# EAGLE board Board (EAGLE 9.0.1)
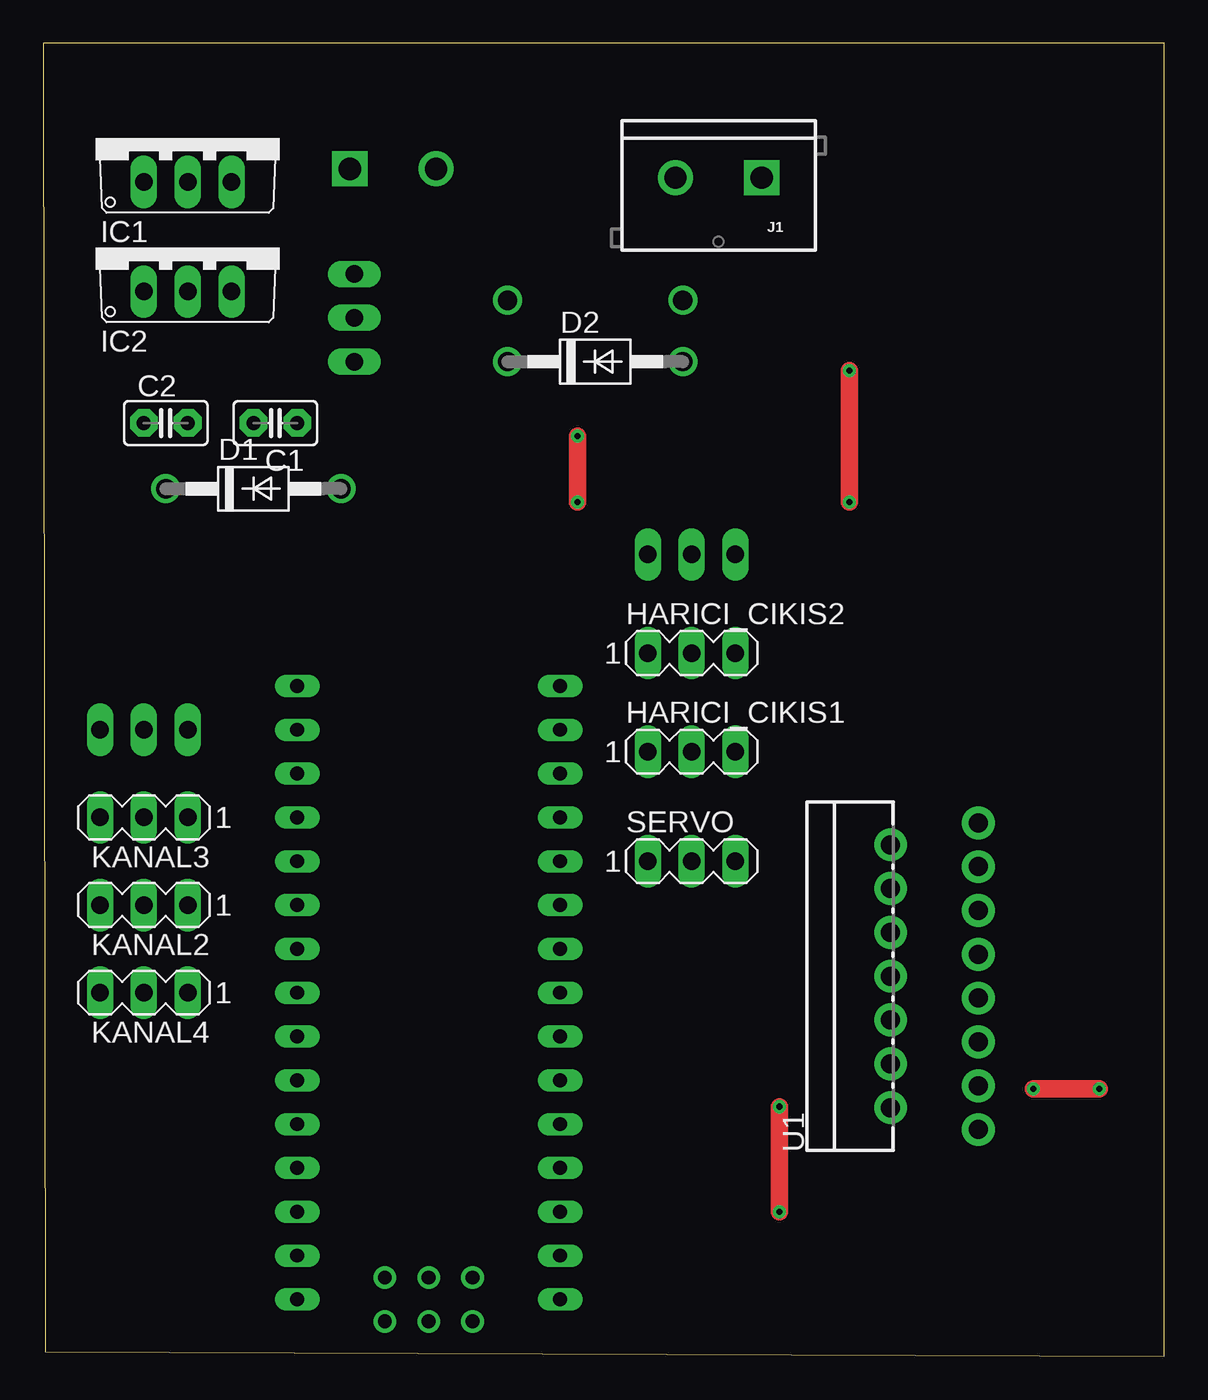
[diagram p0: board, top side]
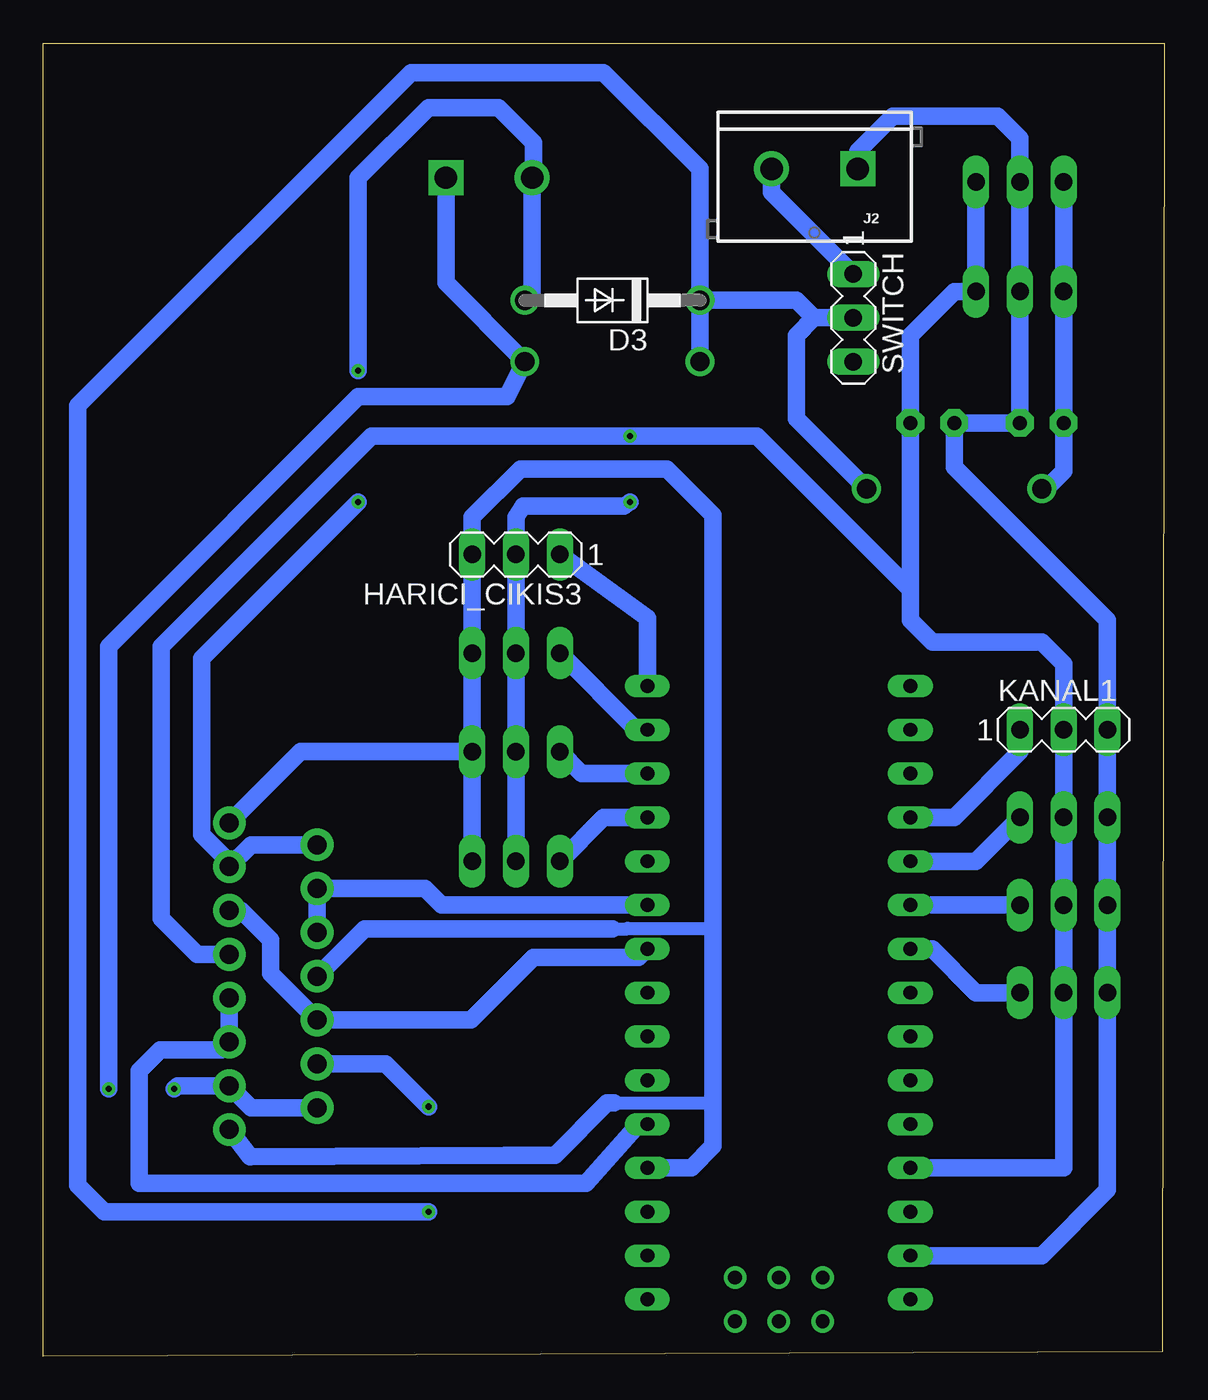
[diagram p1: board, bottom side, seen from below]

Size 65 x 76.12 mm. Coordinates in mm from the lower left corner, seen from the top.
Outline: 0.13,0.25 65,0 65,76.12 0,76.12 0.13,0.25
Copper layers (1*16): Top 0.035mm / dielectric 1.5mm / Bottom 0.035mm
Design rules "default": minimum track width 6mil, minimum drill 0.35mm, track to track 6mil, track to pad 6mil, pad to pad 6mil, via to via 6mil, smd to smd 6mil, copper to edge 40mil, drill to drill 6mil, minimum pad ring 10mil, minimum via ring 8mil, stop-mask expansion 4mil, vias tented up to drill 0mil, thermal gap 10mil

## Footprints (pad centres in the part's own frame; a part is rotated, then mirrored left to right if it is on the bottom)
C2.5-2 = drill 0.813 pad 1.6 octagon: 1 -1.27,0; 2 1.27,0
DO41-10 = drill 1.118: A 5.08,0; C -5.08,0
MA03-1 = drill 1.016 long: 1 -2.54,0; 2 0,0; 3 2.54,0
TO220V = drill 1.016 long: 1 -2.54,-2.54; 2 0,-2.54; 3 2.54,-2.54
SCREWTERMINAL-5MM-2 = drill 1.3 pad 2.032 square: 1 0,0 | drill 1.3 pad 2.032: 2 5,0
MULTIWATT15 = drill 1.1 pad 1.9: 1 -8.95,-2.39; 2 -7.68,2.69; 3 -6.41,-2.39; 4 -5.14,2.69; 5 -3.87,-2.39; 6 -2.6,2.69; 7 -1.33,-2.39; 8 -0.06,2.69; 9 1.21,-2.39; 10 2.48,2.69; 11 3.75,-2.39; 12 5.02,2.69; 13 6.29,-2.39; 14 7.56,2.69; 15 8.83,-2.39
NANO = drill 0.8 long: 3.3V -10.16,24.13; 5V -10.16,-1.27; A0 -10.16,19.05; A1 -10.16,16.51; A2 -10.16,13.97; A3 -10.16,11.43; A4 -10.16,8.89; A5 -10.16,6.35; A6 -10.16,3.81; A7 -10.16,1.27; AREF -10.16,21.59; D2 5.08,1.27; D3 5.08,3.81; D4 5.08,6.35; D5 5.08,8.89; D6 5.08,11.43; D7 5.08,13.97; D8 5.08,16.51; D9 5.08,19.05; D10 5.08,21.59; D11 5.08,24.13; D12 5.08,26.67; D13 -10.16,26.67; GND -10.16,-6.35; GND1 5.08,-1.27; RAW -10.16,-8.89; RST -10.16,-3.81; RST1 5.08,-3.81; RX1 5.08,-6.35; TX0 5.08,-8.89 | drill 0.8: ICSP1 -5.08,-10.16; ICSP2 -5.08,-7.62; ICSP3 -2.54,-10.16; ICSP4 -2.54,-7.62; ICSP5 0,-10.16; ICSP6 0,-7.62

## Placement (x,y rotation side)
C1  0.33uF  [C2.5-2]  13.46,54.1 180 top
C2  0.1uF  [C2.5-2]  7.11,54.1 0 top
D1  1N4004  [DO41-10]  12.19,50.29 0 top
D2  1N4004  [DO41-10]  32,57.66 0 top
D3  1N4004  [DO41-10]  32,61.21 180 bottom
HARICI_CIKIS1  [MA03-1]  37.59,35.05 0 top
HARICI_CIKIS2  [MA03-1]  37.59,40.77 0 top
HARICI_CIKIS3  [MA03-1]  37.59,46.48 180 bottom
IC1  788TV  [TO220V]  8.38,70.61 0 top
IC2  788TV  [TO220V]  8.38,64.26 0 top
J1  [SCREWTERMINAL-5MM-2]  41.66,68.33 180 top
J2  [SCREWTERMINAL-5MM-2]  17.78,68.83 180 bottom
KANAL1  [MA03-1]  5.84,36.32 0 bottom
KANAL2  [MA03-1]  5.84,26.16 180 top
KANAL3  [MA03-1]  5.84,31.24 180 top
KANAL4  [MA03-1]  5.84,21.08 180 top
SERVO  [MA03-1]  37.59,28.7 0 top
SWITCH  [MA03-1]  18.03,60.2 270 bottom
U1  L298  [MULTIWATT15]  51.82,22.1 90 top
U$1  NANO  [NANO]  24.89,12.19 0 top

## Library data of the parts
C1 C2 = capacitor-wima
D1-D3 = diode
HARICI_CIKIS1-HARICI_CIKIS3 KANAL1-KANAL4 SERVO SWITCH = con-lstb; OC_FARNELL: unknown; OC_NEWARK: unknown
IC1 IC2 = linear
J1 J2 = SparkFun-Connectors; SF_SKU: PRT-08432
U1 = SparkFun-IC-Special-Function
U$1 = Arduino

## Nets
A0: KANAL1.1 U$1.A0
A1: KANAL3.1 U$1.A1
A2: KANAL2.1 U$1.A2
A3: KANAL4.1 U$1.A3
D2: U1.5 U1.7 U$1.D2
D3: U$1.D3
D4: U$1.D4
D5: U$1.D5
D6: U1.6 U1.11 U$1.D6
D7: U1.10 U1.12 U$1.D7
D8: U$1.D8
D9: SERVO.1 U$1.D9
D10: HARICI_CIKIS1.1 U$1.D10
D11: HARICI_CIKIS2.1 U$1.D11
D12: HARICI_CIKIS3.1 U$1.D12
DVıN: C2.1 D1.C IC1.1 IC2.1
GND: C1.2 C2.2 IC1.2 IC2.2 J2.1 KANAL1.3 KANAL2.3 KANAL3.3 KANAL4.3 U$1.GND
GND2: HARICI_CIKIS1.3 HARICI_CIKIS2.3 HARICI_CIKIS3.3 SERVO.3 U1.1 U1.8 U1.15 U$1.GND1
N$1: D2.A J1.1 U1.2 U1.3
N$3: J2.2 SWITCH.1
N$4: D3.A J1.2 U1.13 U1.14
VDD: C1.1 HARICI_CIKIS1.2 HARICI_CIKIS2.2 HARICI_CIKIS3.2 IC1.3 IC2.3 KANAL1.2 KANAL2.2 KANAL3.2 KANAL4.2 SERVO.2 U1.9 U$1.5V
VIN: D1.A D2.C D3.C SWITCH.2 U1.4

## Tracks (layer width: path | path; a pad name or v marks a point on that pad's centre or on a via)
A0
  Bottom 1.016: U$1.A0 12.19,31.24 8.38,35.05 KANAL1.1
A1
  Bottom 1.016: U$1.A1 10.92,28.7 KANAL3.1
A2
  Bottom 0.61: 13.46,26.16 U$1.A2
  Bottom 1.016: KANAL2.1 13.46,26.16
A3
  Bottom 0.61: 13.46,23.62 U$1.A3
  Bottom 1.016: KANAL4.1 10.92,21.08 13.46,23.62
D2
  Bottom 1.016: U1.7 U1.5 54.65,17.78 58.21,17.78 59.44,16.55 59.44,10.03 33.53,10.03 30.48,13.46 U$1.D2
D6
  Bottom 1.016: U1.11 53.53,25.85 51.82,24.13 51.82,22.19 U1.6 40.19,19.5 36.58,23.11 30.48,23.11 U$1.D6
D7
  Bottom 1.016: U1.10 U1.12 42.87,27.12 41.91,26.16 U$1.D7
D9
  Bottom 1.016: SERVO.1 32.51,31.24 U$1.D9
D10
  Bottom 1.016: HARICI_CIKIS1.1 33.78,33.78 U$1.D10
D11
  Bottom 1.016: HARICI_CIKIS2.1 30.61,36.32 U$1.D11
D12
  Bottom 1.016: HARICI_CIKIS3.1 29.97,42.8 U$1.D12
DVıN
  Bottom 0.61: IC1.1 IC2.1 5.84,61.47 C2.1 5.84,53.85 | D1.C 6.86,50.29
  Bottom 1.016: IC1.1 5.84,61.47 | IC2.1 5.84,53.85 | C2.1 5.84,51.31 6.86,50.29
GND
  Bottom 1.016: U$1.GND 7.11,5.84 3.3,9.65 KANAL4.3 KANAL2.3 KANAL3.3 KANAL1.3 3.3,42.67 12.19,51.56 C1.2 C2.2 IC2.2 IC1.2 8.38,70.61 9.65,71.88 15.75,71.88 17.78,69.85 J2.1
GND2
  Bottom 0.61: HARICI_CIKIS2.3 40.13,41.4
  Bottom 0.762: 32,24.79 31.14,24.79 31.12,24.81 26.33,24.81 | 31.92,14.69 26.21,14.69 26.16,14.73
  Bottom 1.016: 40.13,41.4 HARICI_CIKIS3.3 40.13,48.64 37.34,51.44 28.83,51.44 26.16,48.77 26.16,24.64 | HARICI_CIKIS2.3 HARICI_CIKIS1.3 | HARICI_CIKIS1.3 SERVO.3 | U$1.GND1 27.43,10.92 26.16,12.19 26.16,14.73 26.16,24.64 | U1.8 46.37,24.79 32,24.79 | U1.15 50.08,35.05 HARICI_CIKIS1.3 | U1.1 53,11.56 38.23,11.66 35.33,11.66 32.3,14.69 31.92,14.69 | 26.16,24.64 26.33,24.81
N$1  (via drill 0.35)
  Top 1.016: v57.4,15.49 v61.21,15.49
  Bottom 1.016: U1.2 52.94,14.42 U1.3 57.21,15.69 v57.4,15.49 | v61.21,15.49 61.21,41.15 46.74,55.63 38.1,55.63 D2.A 41.66,62.23 J1.1
N$3
  Bottom 1.016: SWITCH.1 22.78,67.48 J2.2
N$4  (via drill 0.35)
  Top 1.016: v46.74,49.53 v46.74,57.15
  Bottom 1.016: U1.14 52.94,29.66 U1.13 54.21,28.65 55.82,30.26 55.82,40.45 v46.74,49.53 | v46.74,57.15 46.74,68.33 42.67,72.39 38.61,72.39 36.58,70.36 36.58,68.41 J1.2 36.66,61.64 D3.A
VDD  (via drill 0.35)
  Top 1.016: v30.99,49.53 v30.99,53.34
  Bottom 0.61: HARICI_CIKIS1.2 37.59,40.13 HARICI_CIKIS2.2 HARICI_CIKIS3.2
  Bottom 1.016: IC1.3 IC2.3 12.19,61.72 14.73,59.18 C1.1 14.73,44.45 | U$1.5V 5.84,10.92 KANAL4.2 KANAL2.2 KANAL3.2 KANAL1.2 5.84,40.13 7.11,41.4 13.46,41.4 14.73,42.67 14.73,44.45 | 37.59,40.13 HARICI_CIKIS3.2 37.59,48.64 37.19,49.3 31.34,49.3 v30.99,49.53 | HARICI_CIKIS2.2 HARICI_CIKIS1.2 SERVO.2 | U1.9 56.07,23.31 58.17,25.4 58.17,41.15 45.97,53.34 v30.99,53.34 23.62,53.34 14.73,44.45
VIN  (via drill 0.35)
  Top 1.016: v42.67,14.48 v42.67,8.38
  Bottom 1.016: SWITCH.2 20.32,60.2 | 20.32,60.2 21.34,59.18 21.34,54.36 D1.A | U1.4 45.15,16.96 v42.67,14.48 | v42.67,8.38 61.47,8.38 62.99,9.91 62.99,55.12 43.69,74.42 32.51,74.42 26.92,68.83 D3.C | 20.32,60.2 21.34,61.21 D3.C | D3.C D2.C

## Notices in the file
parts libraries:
SparkFun-IC-Special-Function: Licensing: Creative Commons ShareAlike 4.0 International - https://creativecommons.org/licenses/by-sa/4.0
